FUNCTION_BLOCK FB_DO_IED_LD1_LEDGGIO5_AnOut1 EXTENDS FB_AcsiCommonControllableDataClass
VAR_INPUT
	mxVal: FB_AcsiDATypeAnalogueValue := (fc:=ACSI_FC_MX, TrgOp:=ACSI_TrgOp_dchg, bLinkResult:=THIS^.AddDataToContainer(ipData:=mxVal));
	q: FB_AcsiDATypeQuality := (fc:=ACSI_FC_MX, TrgOp:=ACSI_TrgOp_qchg, bLinkResult:=THIS^.AddDataToContainer(ipData:=q));
	t: FB_AcsiDATypeTimeStamp := (fc:=ACSI_FC_MX, bLinkResult:=THIS^.AddDataToContainer(ipData:=t));
	stSeld: FB_AcsiBATypeBOOLEAN := (fc:=ACSI_FC_MX, TrgOp:=ACSI_TrgOp_dchg, bLinkResult:=THIS^.AddDataToContainer(ipData:=stSeld));
	ctlModel: FB_AcsiDATypeCtlModels := (fc:=ACSI_FC_CF, TrgOp:=ACSI_TrgOp_dchg, eValue:=E_AcsiCtlModels.DirectWithEnhancedSecurity, bLinkResult:=THIS^.AddDataToContainer(ipData:=ctlModel));
	units: FB_AcsiDATypeUnit := (fc:=ACSI_FC_CF, TrgOp:=ACSI_TrgOp_dchg, SIUnit:=(eValue:=E_AcsiSIUnit.Volt), multiplier:=(eValue:=E_AcsiMultiplier.Milli, bPresence:=TRUE), bLinkResult:=THIS^.AddDataToContainer(ipData:=units));
	Oper: FB_AcsiCDC_Oper_AnalogueValue := (fc:=ACSI_FC_CO, bLinkResult:=THIS^.AddDataToContainer(ipData:=Oper));
	
	fbControl: FB_DirectControl := (ipCtrl:=THIS^.AddServerJob(ipEvent:=fbControl, ipCompletion:=fbControl), eType:=E_AcsiCDCType.APC, ipBehVal:=fbIED.IEDLD1.LEDGGIO5.Beh.stVal);
END_VAR
VAR
END_VAR

END_FUNCTION_BLOCK
